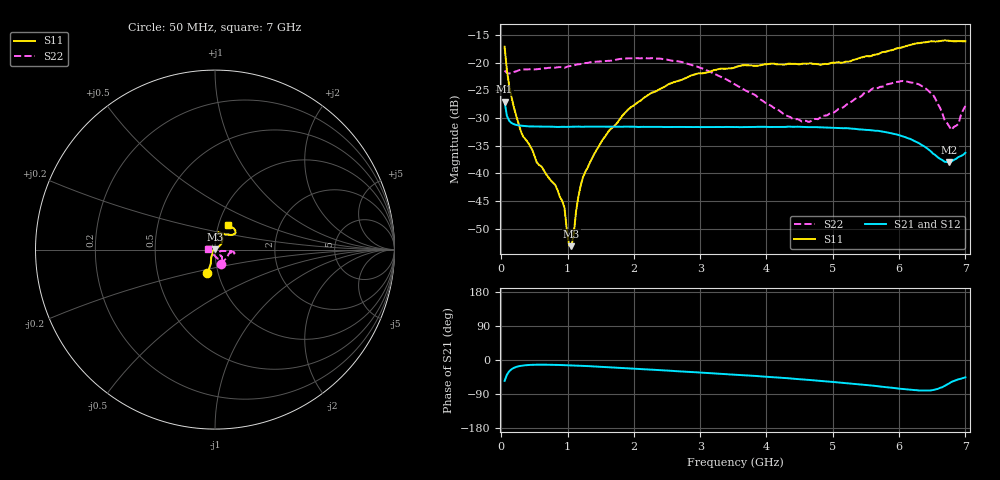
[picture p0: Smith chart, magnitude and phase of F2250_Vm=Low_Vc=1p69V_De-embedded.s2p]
! Integrated Device Technology
! Corporate Headquarters
! 6024 Silver Creek Valley Road
! San Jose, CA 95138  USA
! Phone:  1-408-284-8200
! Toll Free:  1-800-223-1366
! Webpage:  http://www.idt.com/
! Timing and RF Division
! 515 Groton Road, Suite 102
! Westford, MA 01886-6024
! Device:  F2250
! Description: Voltage Variable RF Attenuator
! Frequency:  50.0 -  6000.00 MHz
! Package:  3x3 mm Thin QFN Plastic Package: 16 pin
! Ports:  2 RF, 3 DC
!  Pin  1  = GND
!  Pin  2  = NC
!  Pin  3  = RF1  = Port 1
!  Pin  4  = NC
!  Pin  5  = GND
!  Pin  6  = GND
!  Pin  7  = GND
!  Pin  8  = GND
!  Pin  9  = NC
!  Pin 10  = RF2  = Port 2
!  Pin 11  = NC
!  Pin 12  = GND
!  Pin 13  = GND
!  Pin 14  = VCNTRL
!  Pin 15  = VDD
!  Pin 16  = VMODE
! Vcntrl:  1.690 Volts
! Vmode:  +0.000 Volts
! Vdd:  +3.30  Volts
! Current:  1.187 mA
! Data:  The device was measured on a the F2250 evaluation board which has
!  individual transmission lines to the RF pins.  Data was collected
!  using a calibrated network analyzer.  The evaluation board was
!  de-embedded using a TRL calibration technique.
!  The reference plane is the edge of the package pin.
! Misc:  SN 10
!  Action Tracker AT0258
! Date Measured:  2014-11-26
! Date:  2015-10-15  MJV
! Note:
!  Integrated Device Technology supplies this data as a sample of measured
!  data at the package pin for this product.  Your particular data for this
!  product may vary.
!  Data was taken at 25 degrees C.
!  Integrated Device Technology reserves the right to change this data at anytime.
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# GHz S dB R 50
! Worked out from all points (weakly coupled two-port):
!   201 points, 50 MHz to 7 GHz, reference 50 ohm
!   highest |S21| = -27.09 dB at 50 MHz (marker M1); lowest = -38.0 dB at 6.757 GHz (marker M2)
!   lowest |S11| = -53.2 dB at 1.058 GHz (marker M3), VSWR 1.00, Z = 49.9 + j0.209 ohm
!   |S11| at or under -10 dB: start of sweep to end of sweep
!   |S22| runs from -32.2 to -19.2 dB; largest |S21 - S12| = 0.00015
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0.05  -17.15 -107.9  -27.09 -55.1  -27.09 -55.1  -21.44 -68.2
0.1195  -24.20 -110.7  -30.53 -29.8  -30.53 -29.8  -21.97 -22.5
0.29325  -32.34 -125.5  -31.40 -15.4  -31.39 -15.4  -21.29 -10.9
0.5365  -38.06 -152.4  -31.56 -12.4  -31.55 -12.4  -21.20 -8.0
0.8145  -42.11 173.7  -31.63 -12.9  -31.61 -12.9  -20.94 -10.0
0.9535  -46.26 171.8  -31.62 -13.5  -31.63 -13.5  -20.93 -11.0
1.023  -53.03 136.8  -31.61 -13.9  -31.61 -13.9  -20.66 -10.8
1.05775  -53.17 107.8  -31.60 -14.1  -31.62 -14.1  -20.63 -10.8
1.162  -44.30 47.2  -31.57 -14.9  -31.58 -14.9  -20.32 -12.1
1.2315  -40.73 38.7  -31.61 -15.4  -31.59 -15.4  -20.18 -12.6
1.6485  -32.01 39.8  -31.61 -19.2  -31.58 -19.3  -19.67 -11.8
1.9265  -28.35 40.0  -31.60 -22.1  -31.57 -22.1  -19.24 -11.4
2.37825  -24.87 46.4  -31.62 -26.7  -31.60 -26.7  -19.27 -9.3
3.525  -20.87 72.0  -31.65 -38.8  -31.65 -38.8  -23.96 -7.5
4.39375  -20.25 76.6  -31.61 -49.2  -31.60 -49.2  -30.18 -18.4
4.7065  -20.25 72.1  -31.67 -53.5  -31.65 -53.6  -30.23 -31.2
5.85325  -17.86 40.2  -32.72 -72.6  -32.71 -72.6  -23.85 -52.0
6.40925  -16.34 41.6  -35.38 -80.7  -35.40 -80.7  -24.76 -66.9
6.5135  -16.17 44.2  -36.46 -79.2  -36.41 -79.3  -25.84 -75.5
6.75675  -16.08 50.9  -37.96 -61.6  -37.95 -61.5  -31.53 -117.5
6.89575  -16.13 56.8  -37.06 -50.9  -37.06 -50.8  -31.09 -166.1
7  -16.17 63.0  -36.31 -45.7  -36.30 -45.6  -27.84 172.3
